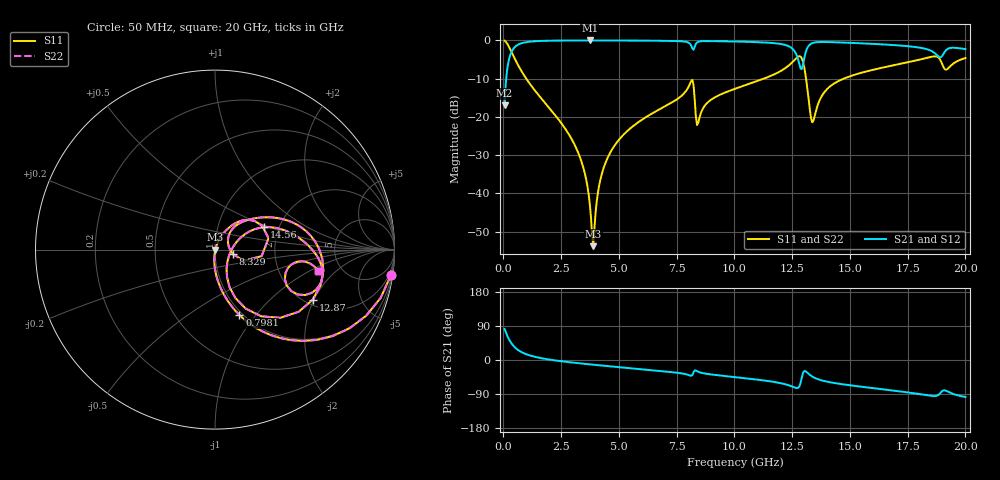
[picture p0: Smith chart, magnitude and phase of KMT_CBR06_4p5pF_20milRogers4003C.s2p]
! Data measured by Modelithics Inc. support@modelithics.com 813-866-6335
! KEMET CBR0603 4.5pF, Pad Width= 0.851mm, Pad Length= 0.64mm, Pad Gap= 0.62mm, 20mil Rogers 4003C substrate Data, January 2022
# hz S ma R 50
! 2 Port Network Data from SP1.SP block
! freq  magS11  angS11  magS21  angS21  magS12  angS12  magS22  angS22
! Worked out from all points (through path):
!   401 points, 50 MHz to 20 GHz, reference 50 ohm
!   highest |S21| = -0.02 dB at 3.741 GHz (marker M1); lowest = -17.0 dB at 50 MHz (marker M2)
!   group delay of S21, straight-line fit = 15.8 ps
!   lowest |S11| = -53.8 dB at 3.89 GHz (marker M3), VSWR 1.00, Z = 50.2 + j0.00663 ohm
!   |S11| at or under -10 dB: 986.5 MHz to 11.27 GHz (10.29 GHz wide, 168 % of centre); 13.1 GHz to 14.73 GHz (1.632 GHz wide, 11.7 % of centre)
!   |S22| runs from -53.8 to -0.1 dB; largest |S21 - S12| = 0
!   S11 on the Smith chart (normalised r, x): 50 MHz: 1, -14; 798.1 MHz: 0.97, -0.83; 8.329 GHz: 1.22, -0.06; 12.87 GHz: 2.19, -1.96; 14.56 GHz: 1.67, +0.46; 20 GHz: 3.38, -1.22
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5e7  0.99 -8.3  0.1411 81.7  0.1411 81.7  0.99 -8.3
2.99375e8  0.7585 -41.6  0.6509 48.4  0.6509 48.4  0.7585 -41.6
7.98125e8  0.3883 -69.6  0.9205 20.3  0.9205 20.3  0.3883 -69.6
3.391625e9  0.02532 -95.2  0.9977 -9.4  0.9977 -9.4  0.02532 -95.2
3.74075e9  0.007167 -85.8  0.9979 -11.6  0.9979 -11.6  0.007167 -85.8
3.890375e9  0.002045 1.8  0.9979 -12.5  0.9979 -12.5  0.002045 1.8
4.189625e9  0.01482 67.8  0.9977 -14.2  0.9977 -14.2  0.01482 67.8
4.6385e9  0.0348 69.6  0.9971 -16.8  0.9971 -16.8  0.0348 69.6
6.73325e9  0.1244 60.0  0.9888 -28.6  0.9888 -28.6  0.1244 60.0
8.12975e9  0.2952 26.7  0.8525 -41.7  0.8525 -41.7  0.2952 26.7
8.32925e9  0.1026 -14.5  0.8995 -27.8  0.8995 -27.8  0.1026 -14.5
8.429e9  0.08328 30.0  0.9565 -30.9  0.9565 -30.9  0.08328 30.0
1.0025e10  0.2331 43.6  0.9669 -45.2  0.9669 -45.2  0.2331 43.6
1.231925e10  0.4611 18.9  0.8474 -66.1  0.8474 -66.1  0.4611 18.9
1.286788e10  0.6119 -27.1  0.4277 -59.6  0.4277 -59.6  0.6119 -27.1
1.311725e10  0.2929 -67.2  0.7475 -31.3  0.7475 -31.3  0.2929 -67.2
1.336662e10  0.08515 -23.9  0.9189 -43.6  0.9189 -43.6  0.08515 -23.9
1.456362e10  0.3 24.5  0.9404 -63.0  0.9404 -63.0  0.3 24.5
1.670825e10  0.4608 9.2  0.8761 -79.4  0.8761 -79.4  0.4608 9.2
1.890275e10  0.5621 -26.7  0.5996 -88.1  0.5996 -88.1  0.5621 -26.7
1.9202e10  0.4188 -14.4  0.7632 -82.2  0.7632 -82.2  0.4188 -14.4
2e10  0.5879 -11.6  0.7691 -97.7  0.7691 -97.7  0.5879 -11.6
